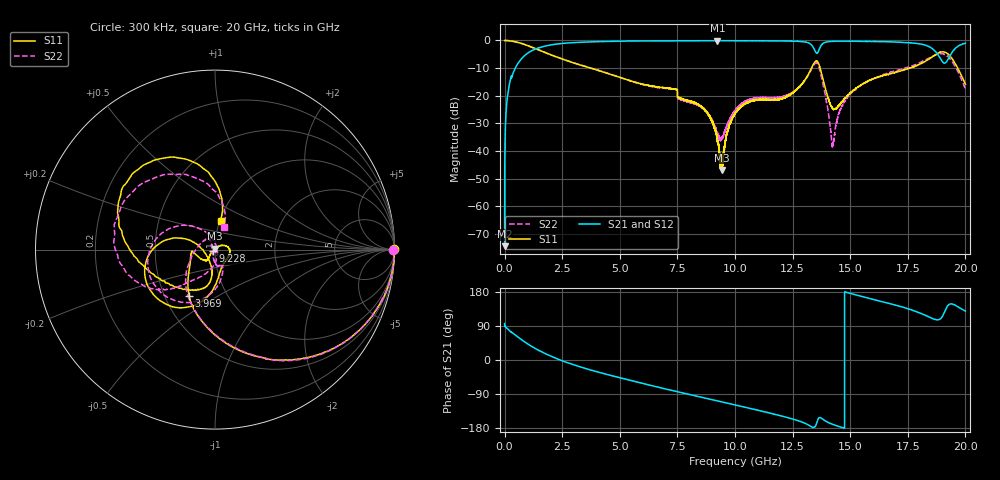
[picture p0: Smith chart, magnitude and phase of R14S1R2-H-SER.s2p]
!{R14S1R2}
!Johanson Technology Inc.
!www.johansontechnology.com
!Test Board Conditions:
!Substrate Type  RO4350B
!Substrate Thickness  20 mil
!Substrate Dk  3.66
!TL Type: GCPW
!TL Trace Width  36 mil
!TL Gap  12 mil
!Electrode orientation  Horizontal
!DUT TOPOLOGY	SERIES
!Mounting Pad LxW  26x36 mil
! Created Wed Nov 25 17:33:21 2020
! 2 Port Network Data from SP1.SP block
! freq  magS11  angS11  magS21  angS21  magS12  angS12  magS22  angS22
# khz S ma R 50
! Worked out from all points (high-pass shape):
!   20001 points, 300 kHz to 20 GHz, reference 50 ohm
!   highest |S21| = -0.07 dB at 9.237 GHz (marker M1); lowest = -74.5 dB at 300 kHz (marker M2)
!   |S21| within 3 dB of the highest: 1.348 GHz to 13.44 GHz (12.09 GHz wide, 164 % of centre); 13.66 GHz to 18.58 GHz (4.919 GHz wide, 30.5 % of centre)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
!   lowest |S11| = -46.9 dB at 9.448 GHz (marker M3), VSWR 1.01, Z = 49.9 + j0.436 ohm
!   |S11| at or under -10 dB: 3.73 GHz to 13.32 GHz (9.59 GHz wide, 112 % of centre); 13.69 GHz to 17.57 GHz (3.877 GHz wide, 24.8 % of centre); 19.66 GHz to end of sweep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
!   |S22| runs from -38.5 to 0.0 dB; largest |S21 - S12| = 0.02
!   S11 on the Smith chart (normalised r, x): 300 kHz: open; 3.969 GHz: 0.66, -0.37; 9.228 GHz: 0.97, -0.02; 20 GHz: 1.01, +0.33
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300  0.9948 0.0  0.0001883 96.5  0.0002679 90.5  0.9935 -0.0
132300  0.9938 -7.6  0.1037 82.3  0.1041 82.2  0.9944 -7.6
504300  0.938 -25.7  0.3397 63.8  0.3405 64.0  0.9369 -25.7
1851300  0.5838 -75.7  0.8048 14.3  0.807 14.4  0.5836 -75.2
3334300  0.3542 -109.1  0.9282 -19.2  0.9284 -19.1  0.3565 -108.5
3969300  0.2946 -119.3  0.9481 -30.3  0.949 -30.3  0.296 -120.6
6667300  0.1438 -161.2  0.9825 -71.8  0.9821 -71.8  0.1408 -160.8
8597300  0.06074 -127.5  0.9885 -99.1  0.9899 -99.0  0.05946 116.7
9228300  0.01559 -148.8  0.9906 -107.8  0.9895 -107.9  0.02043 146.4
9237300  0.0147 -148.7  0.9922 -107.9  0.9886 -108.0  0.02024 149.9
9448300  0.00453 105.3  0.9898 -110.8  0.9908 -110.9  0.01684 -152.8
1.00003e7  0.04796 28.8  0.9881 -118.6  0.9872 -118.6  0.05395 -97.1
1.23543e7  0.102 -67.3  0.9727 -153.2  0.9775 -153.2  0.1069 -67.2
1.33343e7  0.3262 -109.4  0.8182 -176.7  0.8208 -176.9  0.3091 -110.5
1.36723e7  0.34 178.3  0.7199 -151.9  0.7159 -152.2  0.2996 160.2
1.42473e7  0.05797 -160.1  0.9643 -170.1  0.9656 -170.0  0.01299 -1.8
1.49293e7  0.104 -100.9  0.9705 177.0  0.9697 176.9  0.09939 -99.1
1.66673e7  0.2418 -113.7  0.9471 149.5  0.9392 149.4  0.2605 -131.9
1.82003e7  0.4074 -166.8  0.834 119.5  0.8246 119.1  0.4281 -150.8
1.88493e7  0.5984 153.6  0.5193 106.4  0.5218 107.1  0.5651 171.2
1.93073e7  0.5361 109.1  0.5057 147.2  0.512 147.3  0.4775 118.6
2e7  0.1619 79.1  0.8883 129.2  0.8885 129.2  0.1312 68.4
